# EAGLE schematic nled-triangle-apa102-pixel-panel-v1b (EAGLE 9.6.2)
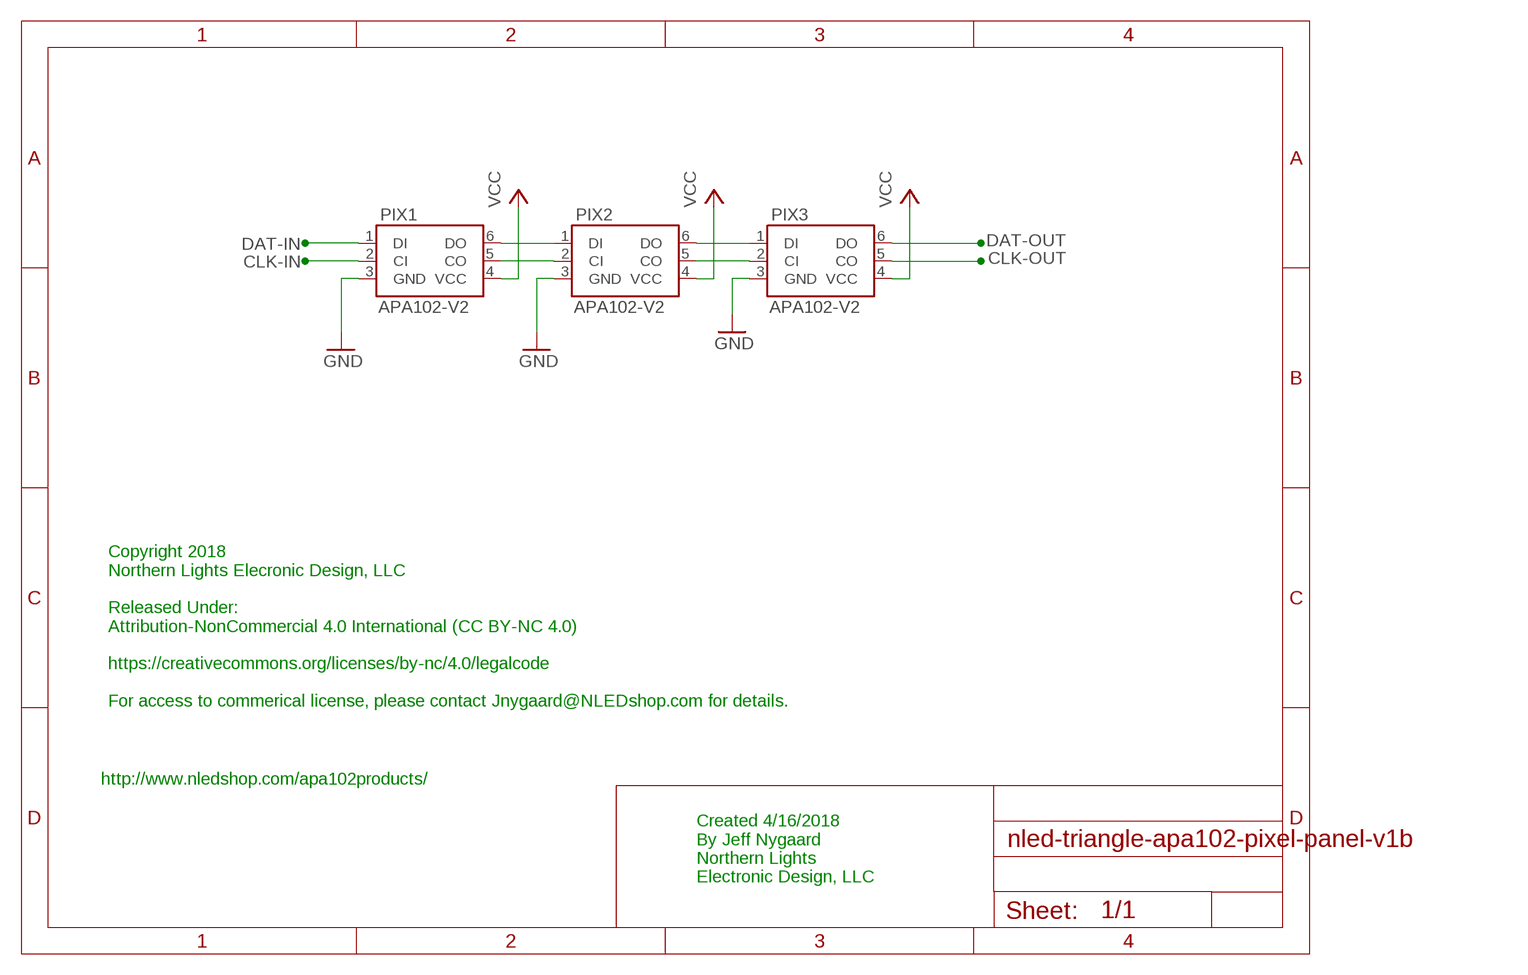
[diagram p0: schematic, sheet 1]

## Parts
PIX1  APA102-V2  [APA102_5050]
PIX2  APA102-V2  [APA102_5050]
PIX3  APA102-V2  [APA102_5050]

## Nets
CLK-IN: PIX1.2(CI)
CLK-OUT: PIX3.5(CO)
DAT-IN: PIX1.1(DI)
DAT-OUT: PIX3.6(DO)
GND: PIX1.3(GND) PIX2.3(GND) PIX3.3(GND)
N$1: PIX1.6(DO) PIX2.1(DI)
N$2: PIX1.5(CO) PIX2.2(CI)
N$6: PIX2.6(DO) PIX3.1(DI)
N$7: PIX2.5(CO) PIX3.2(CI)
VCC: PIX1.4(VCC) PIX2.4(VCC) PIX3.4(VCC)

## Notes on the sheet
- Copyright 2018
  Northern Lights Elecronic Design, LLC
  
  Released Under:
  Attribution-NonCommercial 4.0 International (CC BY-NC 4.0)
  
  https://creativecommons.org/licenses/by-nc/4.0/legalcode
  
  For access to commerical license, please contact Jnygaard@NLEDshop.com for details.
- http://www.nledshop.com/apa102products/
- Created 4/16/2018
  By Jeff Nygaard
  Northern Lights
  Electronic Design, LLC

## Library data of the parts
PIX1-PIX3 = NLED-optoelectric:APA102-V2

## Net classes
0 default: width 0.61 mm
